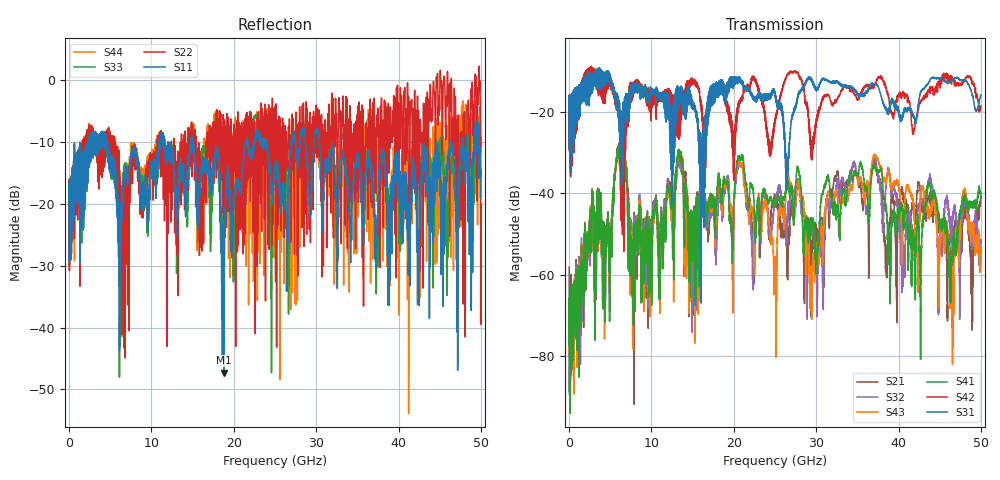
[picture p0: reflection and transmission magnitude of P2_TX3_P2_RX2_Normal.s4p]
!Keysight Technologies,N5225B,MY57041031,A.13.20.10
!Date: Friday, May 31, 2019 11:29:13
!Correction: S11(Full 4 Port(1,2,3,4))
!S12(Full 4 Port(1,2,3,4))
!S13(Full 4 Port(1,2,3,4))
!S14(Full 4 Port(1,2,3,4))
!S21(Full 4 Port(1,2,3,4))
!S22(Full 4 Port(1,2,3,4))
!S23(Full 4 Port(1,2,3,4))
!S24(Full 4 Port(1,2,3,4))
!S31(Full 4 Port(1,2,3,4))
!S32(Full 4 Port(1,2,3,4))
!S33(Full 4 Port(1,2,3,4))
!S34(Full 4 Port(1,2,3,4))
!S41(Full 4 Port(1,2,3,4))
!S42(Full 4 Port(1,2,3,4))
!S43(Full 4 Port(1,2,3,4))
!S44(Full 4 Port(1,2,3,4))
!S4P File: Measurements: <S11,S12,S13,S14>,
!<S21,S22,S23,S24>,
!<S31,S32,S33,S34>,
!<S41,S42,S43,S44>:
# Hz S  dB  R 50.0
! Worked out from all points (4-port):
!   5000 points, 10 MHz to 50 GHz, reference 50 ohm
!   strongest paths, dB at 10 MHz, 12.51 GHz, 25.01 GHz, 37.51 GHz, 50 GHz:
!     S31: -19.5, -42.4, -16.0, -13.6, -15.6
!     S42: -19.5, -15.9, -21.9, -11.5, -18.5
!     S41: -67.9, -40.9, -42.2, -34.2, -41.0
!     S43: -66.5, -43.5, -56.6, -31.4, -53.2
!     S32: -68.6, -42.8, -42.5, -35.7, -51.9
!     S21: -58.2, -40.6, -41.4, -36.7, -41.1
!   lowest |S11| = -47.3 dB at 18.82 GHz (marker M1), VSWR 1.01, Z = 49.6 + j0.123 ohm
!   |S11| at or under -10 dB: 4.63 GHz to 10.95 GHz (6.318 GHz wide, 81.1 % of centre); 15.04 GHz to 21.46 GHz (6.423 GHz wide, 35.2 % of centre); 30.38 GHz to 44.61 GHz (14.22 GHz wide, 37.9 % of centre)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
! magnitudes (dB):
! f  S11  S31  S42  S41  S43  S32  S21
! 10 MHz  -19.6  -19.5  -19.5  -67.9  -66.5  -68.6  -58.2
! 6.04 GHz  -22.0  -18.2  -19.0  -28.1  -29.0  -28.3  -27.6
! 7.81 GHz  -10.8  -13.1  -12.7  -57.9  -54.9  -56.1  -60.2
! 18.82 GHz  -47.3  -13.3  -16.1  -36.6  -37.4  -38.6  -38.2
! 37.17 GHz  -23.7  -13.0  -13.0  -33.8  -30.6  -31.5  -32.5
! 46.25 GHz  -11.8  -12.5  -12.0  -62.9  -58.0  -46.8  -55.2
! 50 GHz  -15.5  -15.6  -18.5  -41.0  -53.2  -51.9  -41.1
